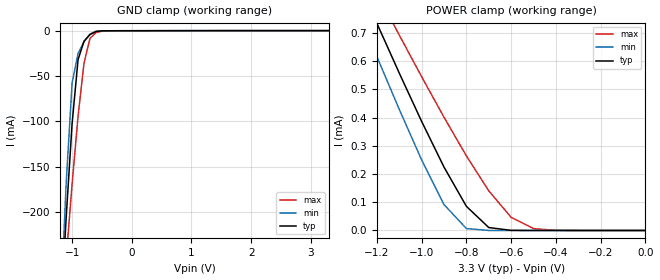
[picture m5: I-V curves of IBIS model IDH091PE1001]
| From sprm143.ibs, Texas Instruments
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[Model]   IDH091PE1001
| Input with pulldown
Model_type   Input
Polarity   Non-Inverting
| signals   A, Y
Vinl = 0.8V
Vinh = 2.0V
|   typ   min   max
C_comp   1.5797p   1.5046p   1.7659p
|   typ   min   max
[Temperature Range]   25   -40   125
|   typ   min   max
[Voltage Range]   3.30V   3.00V   3.60V
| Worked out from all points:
|   GND clamp passes 1 mA (typ) near -0.60 V on its own axis
|   POWER clamp passes 1 mA (typ) near -1.35 V on its own axis
[GND_clamp]
|   Voltage   I(typ)   I(min)   I(max)
-3.3V     -3.036A    -3.942A    -2.292A
-1.2V     -323.1mA   -318.8mA   -337.7mA
-1.1V     -206.9mA   -169.3mA   -251.7mA
-1V       -102.5mA   -57.62mA   -169.3mA
-900mV    -31.82mA   -25.05mA   -94.2mA
-800mV    -11.49mA   -12.18mA   -35.59mA
-700mV    -4.254mA   -3.657mA   -8.535mA
-600mV    -873.9uA   -493.6uA   -2.077mA
-500mV    -120.6uA   -88.85uA   -393.8uA
-400mV    -40.17uA   -55.66uA   -66.09uA
3.3V      100.3uA    176.6uA    51.97uA
[POWER_clamp]
|   Voltage   I(typ)   I(min)   I(max)
-3.3V     4.645mA    4.788mA    4.153mA
-1.3V     913.9uA    807.7uA    995.7uA
-1.2V     734.6uA    616.6uA    843.4uA
-1.1V     558.3uA    429.5uA    693uA
-1V       386.8uA    250.3uA    545.2uA
-900mV    224.7uA    91.79uA    401.4uA
-800mV    85.58uA    6.841uA    264.4uA
-700mV    10.38uA    74.43nA    140.5uA
-600mV    332.6nA    977pA      46.51uA
-500mV    8.571nA    266.4pA    6.514uA
-400mV    532.9pA    222pA      470.9nA
0V        266.4pA    177.6pA    2.798nA
